(* Logix 5000 AddOnInstructionDefinition export Banner_R95C8UI_PD_v4; software revision 33.00 *)

TYPE Banner_R95C_8UI_PDI0_v4 :
STRUCT
   Value : DINT[9];
END_STRUCT
END_TYPE

TYPE Banner_R95C_8UI_PDI1_v4 :
STRUCT
   Device : Banner_R95C_8UI_Sensor_Profile_v4[9];
END_STRUCT
END_TYPE

TYPE Banner_R95C_8UI_PDIO_v4 :
STRUCT
   Set0 : Banner_R95C_8UI_PDI0_v4;
   Set1 : Banner_R95C_8UI_PDI1_v4;
   DTI : SINT[32];
END_STRUCT
END_TYPE

TYPE Banner_R95C_8UI_Sensor_Profile_v4 :
STRUCT
   Value : DINT;
   Scale : INT;
   Switching_Signal : SINT;
END_STRUCT
END_TYPE

ADD_ON_INSTRUCTION Banner_R95C8UI_PD_v4   (* revision 4.0, vendor Banner Engineering *)
// AOI that used with the R95C-8UI-KQ hub.
VAR_IN_OUT
   PD : Banner_R95C_8UI_PDIO_v4; {required}
END_VAR
VAR_INPUT
   PDI_Config : SINT; {required}
   Byte_Swap : BOOL; {required}
END_VAR
VAR
   TempIn : SINT[32]; {access None}
END_VAR

ROUTINE Logic   (* ladder *)
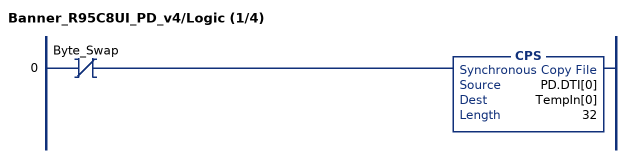
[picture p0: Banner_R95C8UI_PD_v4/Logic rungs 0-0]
   0: XIO(Byte_Swap)CPS(PD.DTI[0],TempIn[0],32);
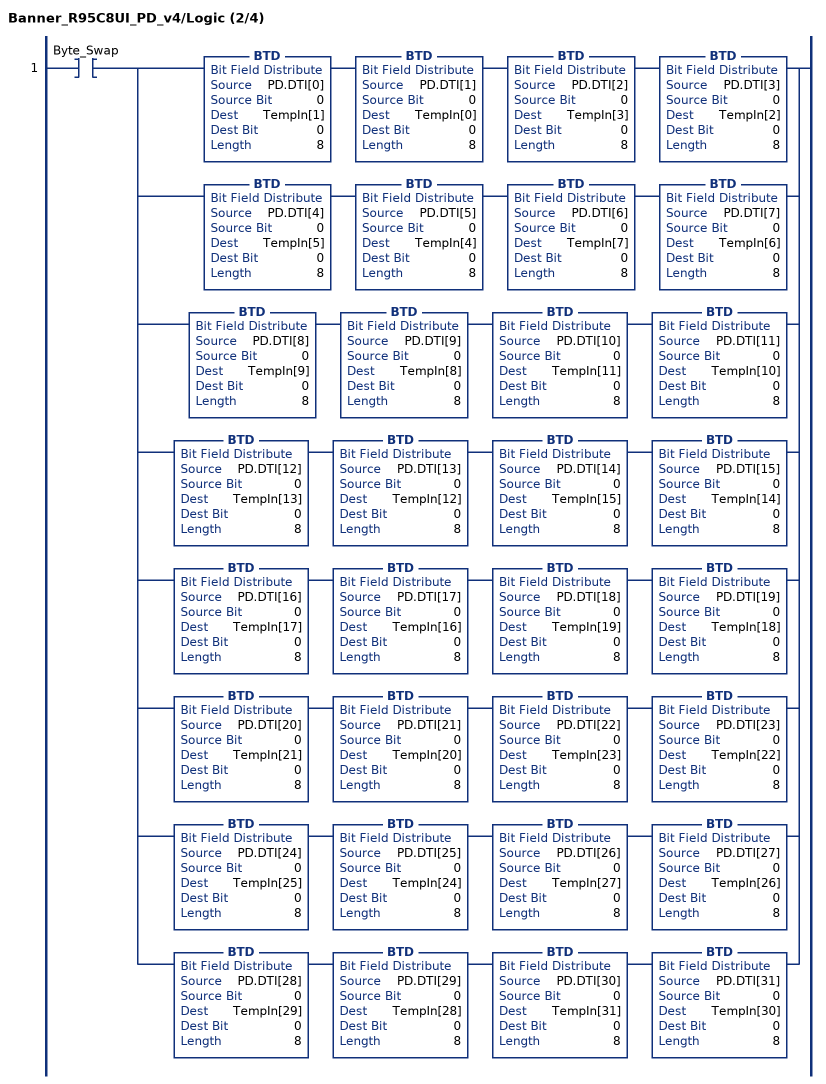
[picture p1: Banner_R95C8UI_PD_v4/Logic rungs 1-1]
   1: XIC(Byte_Swap)[BTD(PD.DTI[0],0,TempIn[1],0,8) BTD(PD.DTI[1],0,TempIn[0],0,8) BTD(PD.DTI[2],0,TempIn[3],0,8) BTD(PD.DTI[3],0,TempIn[2],0,8) ,BTD(PD.DTI[4],0,TempIn[5],0,8) BTD(PD.DTI[5],0,TempIn[4],0,8) BTD(PD.DTI[6],0,TempIn[7],0,8) BTD(PD.DTI[7],0,TempIn[6],0,8) ,BTD(PD.DTI[8],0,TempIn[9],0,8) BTD(PD.DTI[9],0,TempIn[8],0,8) BTD(PD.DTI[10],0,TempIn[11],0,8) BTD(PD.DTI[11],0,TempIn[10],0,8) ,BTD(PD.DTI[12],0,TempIn[13],0,8) BTD(PD.DTI[13],0,TempIn[12],0,8) BTD(PD.DTI[14],0,TempIn[15],0,8) BTD(PD.DTI[15],0,TempIn[14],0,8) ,BTD(PD.DTI[16],0,TempIn[17],0,8) BTD(PD.DTI[17],0,TempIn[16],0,8) BTD(PD.DTI[18],0,TempIn[19],0,8) BTD(PD.DTI[19],0,TempIn[18],0,8) ,BTD(PD.DTI[20],0,TempIn[21],0,8) BTD(PD.DTI[21],0,TempIn[20],0,8) BTD(PD.DTI[22],0,TempIn[23],0,8) BTD(PD.DTI[23],0,TempIn[22],0,8) ,BTD(PD.DTI[24],0,TempIn[25],0,8) BTD(PD.DTI[25],0,TempIn[24],0,8) BTD(PD.DTI[26],0,TempIn[27],0,8) BTD(PD.DTI[27],0,TempIn[26],0,8) ,BTD(PD.DTI[28],0,TempIn[29],0,8) BTD(PD.DTI[29],0,TempIn[28],0,8) BTD(PD.DTI[30],0,TempIn[31],0,8) BTD(PD.DTI[31],0,TempIn[30],0,8) ];
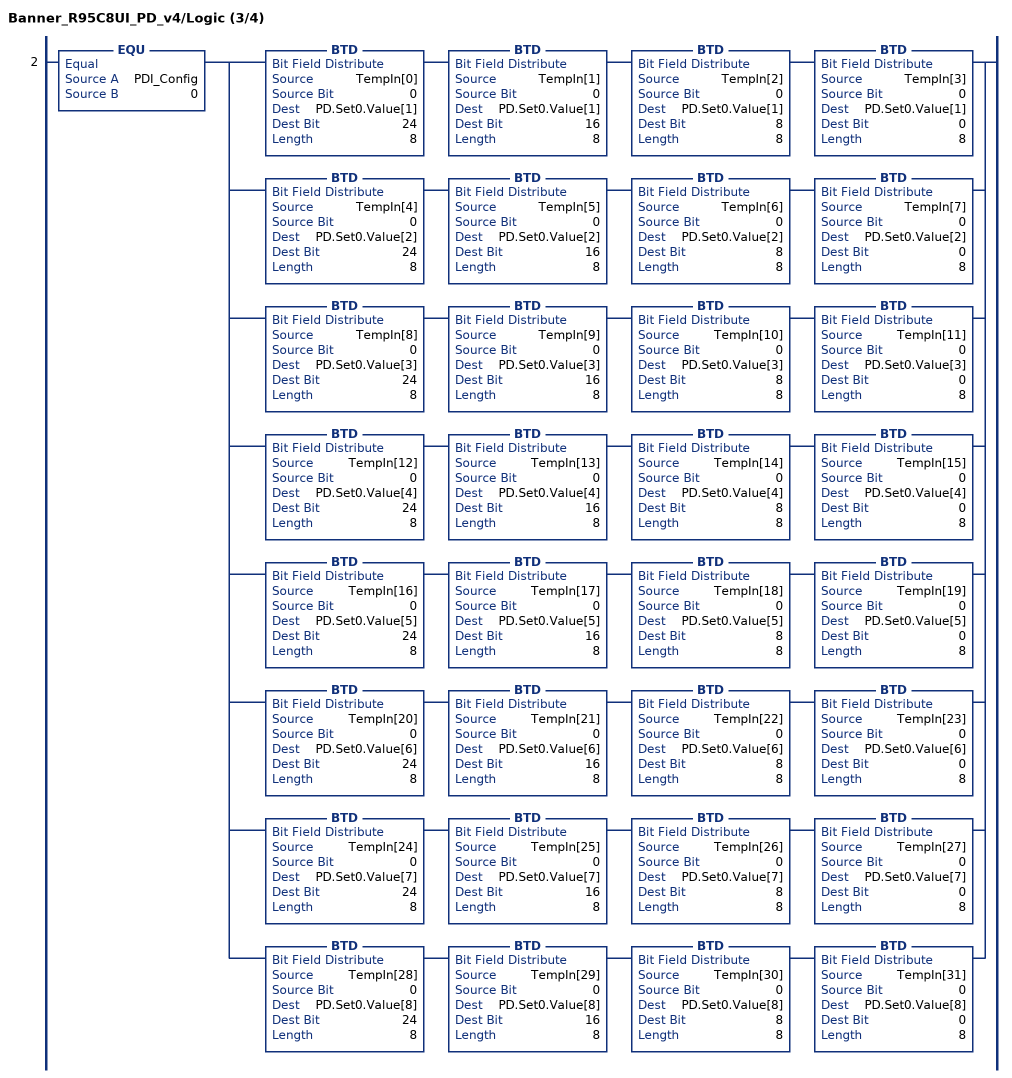
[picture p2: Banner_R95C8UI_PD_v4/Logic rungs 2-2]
   2: EQU(PDI_Config,0)[BTD(TempIn[0],0,PD.Set0.Value[1],24,8) BTD(TempIn[1],0,PD.Set0.Value[1],16,8) BTD(TempIn[2],0,PD.Set0.Value[1],8,8) BTD(TempIn[3],0,PD.Set0.Value[1],0,8) ,BTD(TempIn[4],0,PD.Set0.Value[2],24,8) BTD(TempIn[5],0,PD.Set0.Value[2],16,8) BTD(TempIn[6],0,PD.Set0.Value[2],8,8) BTD(TempIn[7],0,PD.Set0.Value[2],0,8) ,BTD(TempIn[8],0,PD.Set0.Value[3],24,8) BTD(TempIn[9],0,PD.Set0.Value[3],16,8) BTD(TempIn[10],0,PD.Set0.Value[3],8,8) BTD(TempIn[11],0,PD.Set0.Value[3],0,8) ,BTD(TempIn[12],0,PD.Set0.Value[4],24,8) BTD(TempIn[13],0,PD.Set0.Value[4],16,8) BTD(TempIn[14],0,PD.Set0.Value[4],8,8) BTD(TempIn[15],0,PD.Set0.Value[4],0,8) ,BTD(TempIn[16],0,PD.Set0.Value[5],24,8) BTD(TempIn[17],0,PD.Set0.Value[5],16,8) BTD(TempIn[18],0,PD.Set0.Value[5],8,8) BTD(TempIn[19],0,PD.Set0.Value[5],0,8) ,BTD(TempIn[20],0,PD.Set0.Value[6],24,8) BTD(TempIn[21],0,PD.Set0.Value[6],16,8) BTD(TempIn[22],0,PD.Set0.Value[6],8,8) BTD(TempIn[23],0,PD.Set0.Value[6],0,8) ,BTD(TempIn[24],0,PD.Set0.Value[7],24,8) BTD(TempIn[25],0,PD.Set0.Value[7],16,8) BTD(TempIn[26],0,PD.Set0.Value[7],8,8) BTD(TempIn[27],0,PD.Set0.Value[7],0,8) ,BTD(TempIn[28],0,PD.Set0.Value[8],24,8) BTD(TempIn[29],0,PD.Set0.Value[8],16,8) BTD(TempIn[30],0,PD.Set0.Value[8],8,8) BTD(TempIn[31],0,PD.Set0.Value[8],0,8) ];
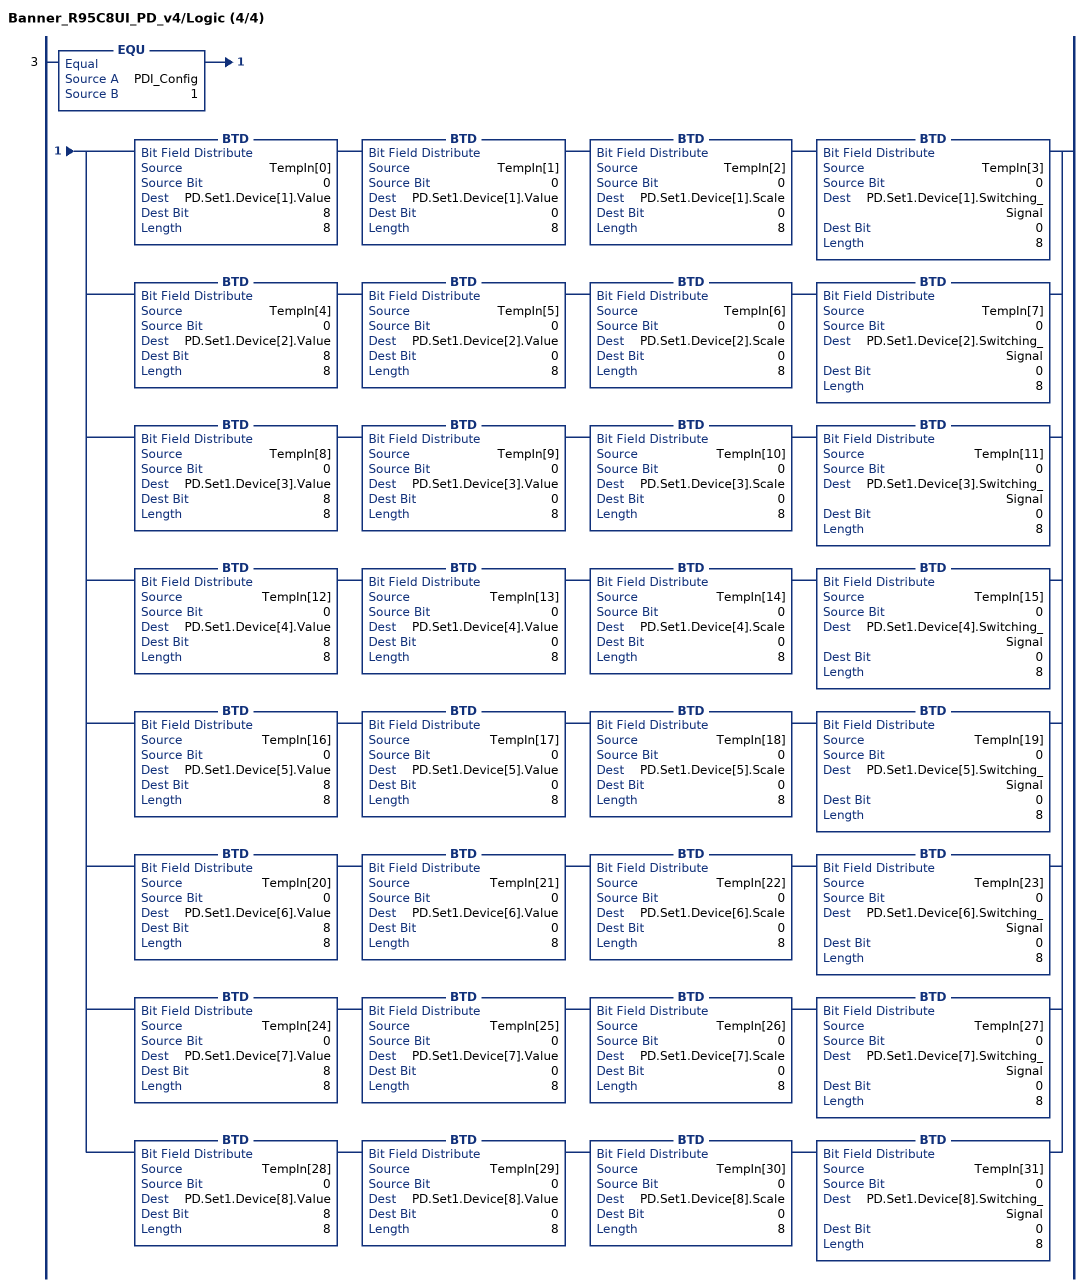
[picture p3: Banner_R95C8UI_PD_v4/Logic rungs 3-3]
   3: EQU(PDI_Config,1)[BTD(TempIn[0],0,PD.Set1.Device[1].Value,8,8) BTD(TempIn[1],0,PD.Set1.Device[1].Value,0,8) BTD(TempIn[2],0,PD.Set1.Device[1].Scale,0,8) BTD(TempIn[3],0,PD.Set1.Device[1].Switching_Signal,0,8) ,BTD(TempIn[4],0,PD.Set1.Device[2].Value,8,8) BTD(TempIn[5],0,PD.Set1.Device[2].Value,0,8) BTD(TempIn[6],0,PD.Set1.Device[2].Scale,0,8) BTD(TempIn[7],0,PD.Set1.Device[2].Switching_Signal,0,8) ,BTD(TempIn[8],0,PD.Set1.Device[3].Value,8,8) BTD(TempIn[9],0,PD.Set1.Device[3].Value,0,8) BTD(TempIn[10],0,PD.Set1.Device[3].Scale,0,8) BTD(TempIn[11],0,PD.Set1.Device[3].Switching_Signal,0,8) ,BTD(TempIn[12],0,PD.Set1.Device[4].Value,8,8) BTD(TempIn[13],0,PD.Set1.Device[4].Value,0,8) BTD(TempIn[14],0,PD.Set1.Device[4].Scale,0,8) BTD(TempIn[15],0,PD.Set1.Device[4].Switching_Signal,0,8) ,BTD(TempIn[16],0,PD.Set1.Device[5].Value,8,8) BTD(TempIn[17],0,PD.Set1.Device[5].Value,0,8) BTD(TempIn[18],0,PD.Set1.Device[5].Scale,0,8) BTD(TempIn[19],0,PD.Set1.Device[5].Switching_Signal,0,8) ,BTD(TempIn[20],0,PD.Set1.Device[6].Value,8,8) BTD(TempIn[21],0,PD.Set1.Device[6].Value,0,8) BTD(TempIn[22],0,PD.Set1.Device[6].Scale,0,8) BTD(TempIn[23],0,PD.Set1.Device[6].Switching_Signal,0,8) ,BTD(TempIn[24],0,PD.Set1.Device[7].Value,8,8) BTD(TempIn[25],0,PD.Set1.Device[7].Value,0,8) BTD(TempIn[26],0,PD.Set1.Device[7].Scale,0,8) BTD(TempIn[27],0,PD.Set1.Device[7].Switching_Signal,0,8) ,BTD(TempIn[28],0,PD.Set1.Device[8].Value,8,8) BTD(TempIn[29],0,PD.Set1.Device[8].Value,0,8) BTD(TempIn[30],0,PD.Set1.Device[8].Scale,0,8) BTD(TempIn[31],0,PD.Set1.Device[8].Switching_Signal,0,8) ];
END_ROUTINE
END_ADD_ON_INSTRUCTION
